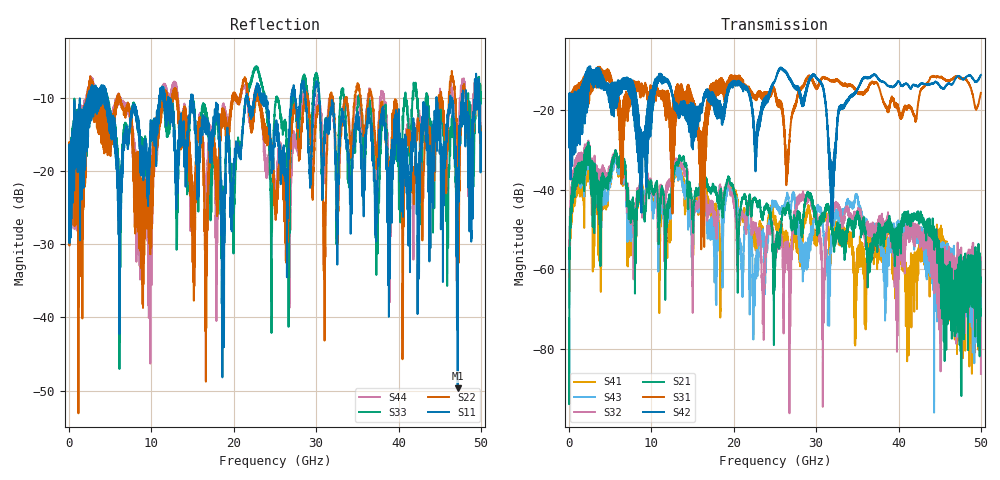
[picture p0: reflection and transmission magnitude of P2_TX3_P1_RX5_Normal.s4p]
!Keysight Technologies,N5225B,MY57041031,A.13.20.10
!Date: Friday, May 31, 2019 11:21:37
!Correction: S11(Full 4 Port(1,2,3,4))
!S12(Full 4 Port(1,2,3,4))
!S13(Full 4 Port(1,2,3,4))
!S14(Full 4 Port(1,2,3,4))
!S21(Full 4 Port(1,2,3,4))
!S22(Full 4 Port(1,2,3,4))
!S23(Full 4 Port(1,2,3,4))
!S24(Full 4 Port(1,2,3,4))
!S31(Full 4 Port(1,2,3,4))
!S32(Full 4 Port(1,2,3,4))
!S33(Full 4 Port(1,2,3,4))
!S34(Full 4 Port(1,2,3,4))
!S41(Full 4 Port(1,2,3,4))
!S42(Full 4 Port(1,2,3,4))
!S43(Full 4 Port(1,2,3,4))
!S44(Full 4 Port(1,2,3,4))
!S4P File: Measurements: <S11,S12,S13,S14>,
!<S21,S22,S23,S24>,
!<S31,S32,S33,S34>,
!<S41,S42,S43,S44>:
# Hz S  dB  R 50.0
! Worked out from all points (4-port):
!   5000 points, 10 MHz to 50 GHz, reference 50 ohm
!   strongest paths, dB at 10 MHz, 12.51 GHz, 25.01 GHz, 37.51 GHz, 50 GHz:
!     S42: -19.6, -15.6, -12.6, -12.1, -11.1
!     S31: -19.6, -43.7, -16.0, -13.6, -15.6
!     S21: -72.3, -39.4, -56.3, -52.1, -70.0
!     S32: -61.1, -36.5, -56.0, -47.8, -86.3
!     S43: -57.8, -40.7, -44.0, -50.3, -72.9
!     S41: -59.6, -43.0, -48.0, -58.3, -64.5
!   lowest |S11| = -49.7 dB at 47.18 GHz (marker M1), VSWR 1.01, Z = 50.3 - j0.106 ohm
!   |S11| at or under -10 dB: 4.63 GHz to 10.95 GHz (6.317 GHz wide, 81.1 % of centre); 15.04 GHz to 21.47 GHz (6.425 GHz wide, 35.2 % of centre); 30.38 GHz to 44.61 GHz (14.23 GHz wide, 37.9 % of centre)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
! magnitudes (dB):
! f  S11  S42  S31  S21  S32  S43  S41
! 10 MHz  -19.1  -19.6  -19.6  -72.3  -61.1  -57.8  -59.6
! 2.3 GHz  -12.6  -16.4  -16.9  -28.3  -27.7  -29.0  -29.3
! 23.58 GHz  -10.1  -19.4  -15.6  -45.6  -66.0  -51.8  -52.1
! 29.79 GHz  -9.5  -11.1  -13.5  -44.7  -44.9  -47.2  -51.1
! 31.93 GHz  -10.6  -38.1  -12.4  -49.6  -45.3  -49.3  -51.8
! 47.18 GHz  -49.7  -11.4  -11.4  -69.9  -53.3  -62.0  -77.8
! 50 GHz  -15.6  -11.1  -15.6  -70.0  -86.3  -72.9  -64.5
